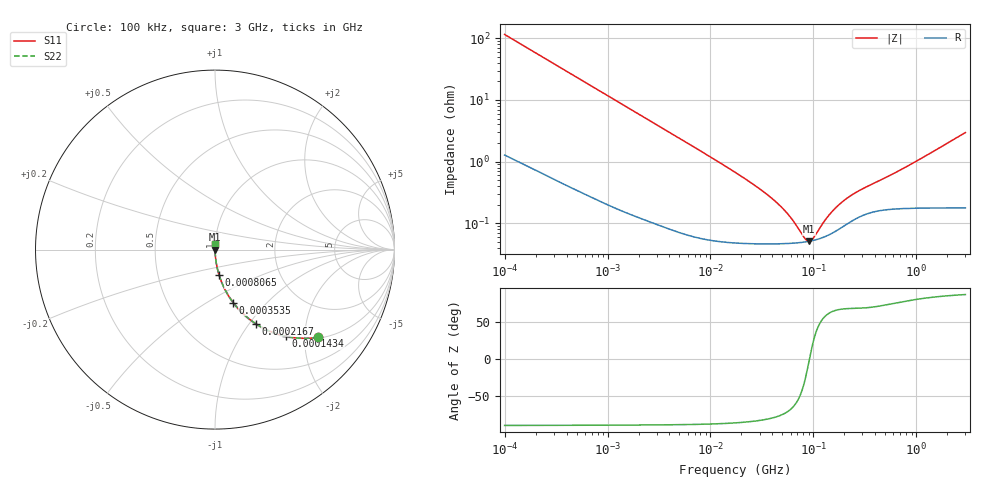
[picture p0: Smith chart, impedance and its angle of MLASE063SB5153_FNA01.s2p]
! MLASE063SB5153_FNA01  S-PARAMETER MODEL  ( Standard Model )
! Model Generated by TAIYO YUDEN Corporation (http://www.ty-top.com)
! Version 1.0
! TAIYO YUDEN Control No. 230906
! Copyright(c) 2018 TAIYO YUDEN CO.,LTD. All Rights Reserved.
! Product Description (link to TY-COMPAS)
! https://ds.yuden.co.jp/TYCOMPAS/or/detail?pn=MLASE063SB5153KFNA01&u=M
! Products Name : Multilayer Ceramic Capacitors
! Characteristics :
!  Capacitance : 0.015 [uF] , Rated Voltage : 16 [V] , TCC : X5R
!  Case Size : 0.6 x 0.3 / 0.024 x 0.012 [mm/inch] , Thickness : 0.3 / 0.012 [mm/inch]
!  (Conditions: Temperature = 25 [degC] , DC Bias Voltage = 0 [V])
! External Node Assignments :
!  1  o---| |---o  2
! GND o---------o GND
! Frequency Range : 100kHz  -  3GHz  [ 401 STEP ]
# MHZ S RI R 50
! Freq[MHz].  S11 Real  S11 Imag  S21 Real  S21 Imag  S12 Real  S12 Imag  S22 Real  S22 Imag
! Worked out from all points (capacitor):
!   401 points, 100 kHz to 3 GHz, reference 50 ohm
!   read as one part in series: C = 13.7 nF near 105.3 kHz
!   lowest |Z| = 50.9 mohm at 90.14 MHz (marker M1)
!   series resonance near 91.66 MHz, so ESL is about 220 pH
!   S11 on the Smith chart (normalised r, x): 100 kHz: 1.03, -2.31; 143.4 kHz: 1.02, -1.62; 216.7 kHz: 1.01, -1.07; 353.5 kHz: 1.01, -0.66; 806.5 kHz: 1.00, -0.29; 3 GHz: 1.00, +0.06
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0.1  0.5716 -0.4894  0.4284 0.4894  0.4284 0.4894  0.5716 -0.4894
0.14345  0.3964 -0.4833  0.6036 0.4833  0.6036 0.4833  0.3964 -0.4833
0.216663  0.2266 -0.4124  0.7734 0.4124  0.7734 0.4124  0.2266 -0.4124
0.353547  0.1016 -0.2953  0.8984 0.2953  0.8984 0.2953  0.1016 -0.2953
0.562235  0.0444 -0.1986  0.9556 0.1986  0.9556 0.1986  0.0444 -0.1986
0.806524  0.023 -0.1421  0.977 0.1421  0.977 0.1421  0.023 -0.1421
1.497078  0.00765 -0.0782  0.9923 0.0782  0.9923 0.0782  0.00765 -0.0782
3.161081  0.00233 -0.0375  0.9977 0.0375  0.9977 0.0375  0.00233 -0.0375
17.7727  0.000517 -0.00651  0.9995 0.00651  0.9995 0.00651  0.000517 -0.00651
30.53531  0.000473 -0.00351  0.9995 0.00351  0.9995 0.00351  0.000473 -0.00351
44.94634  0.000466 -0.00204  0.9995 0.00204  0.9995 0.00204  0.000466 -0.00204
59.67813  0.000471 -0.00117  0.9995 0.00117  0.9995 0.00117  0.000471 -0.00117
83.42988  0.000496 -0.000249  0.9995 0.000249  0.9995 0.000249  0.000496 -0.000249
90.13636  0.000507 -4.42e-05  0.9995 4.42e-05  0.9995 4.42e-05  0.000507 -4.42e-05
97.38194  0.00052 0.000161  0.9995 -0.000161  0.9995 -0.000161  0.00052 0.000161
139.694  0.00064 0.00114  0.9994 -0.00114  0.9994 -0.00114  0.00064 0.00114
163.0551  0.000735 0.00158  0.9993 -0.00158  0.9993 -0.00158  0.000735 0.00158
190.323  0.000864 0.00203  0.9991 -0.00203  0.9991 -0.00203  0.000864 0.00203
273.0175  0.00124 0.00307  0.9988 -0.00307  0.9988 -0.00307  0.00124 0.00307
547.5153  0.0017 0.00564  0.9983 -0.00564  0.9983 -0.00564  0.0017 0.00564
965.2458  0.00184 0.00961  0.9982 -0.00961  0.9982 -0.00961  0.00184 0.00961
3000  0.00264 0.0294  0.9974 -0.0294  0.9974 -0.0294  0.00264 0.0294
